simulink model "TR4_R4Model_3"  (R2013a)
settings: Solver=ode23tb  StartTime=0  StopTime=1  FixedStep=1e-4
PreLoadFcn:
  | warning('off','sm:sli:setup:compile:LocalSolverNotSupported')
InitFcn:
  |  SimParam.IC = SM2_InitCondConstrFnc(RawParam,IC);
model workspace (MAT data in the model file):
  handle : class17 (value not decoded)
  handle : class17 (value not decoded)
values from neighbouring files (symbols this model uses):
  RawParam = RobotParamGather(ParamLib)    [main_TR4.m]    (also in DeltaModelMain_v2.m; main_TimeSimulation.m; MGI.m = y)
libraries: SM2_BallJointPartsLib x8, SM2_ForeArmPartsLib x8, SM2_ArmPartsLib x4, SM2_MotorPartsLib x4, ElecDriverLib x1, SM2_FramePartsLib x1, SM2_ToolPartsLib x1

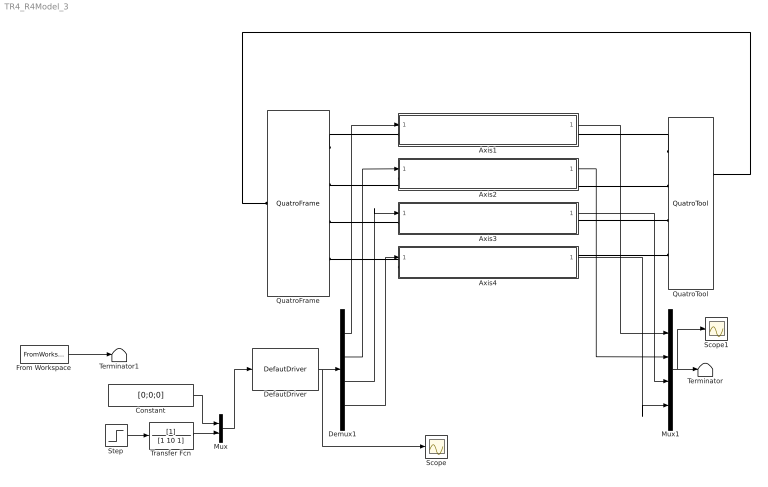
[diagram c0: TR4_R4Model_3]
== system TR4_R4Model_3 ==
  Axis1 : Subsystem
  Axis2 : Subsystem
  Axis3 : Subsystem
  Axis4 : Subsystem
  Constant : Constant  Value=[0;0;0]
  DefautDriver : ElecDriverLib/DefautDriver  VariantControl=driverVarDefault
  Demux1 : Demux
  From Workspace : FromWorkspace  VariableName=simin  SampleTime=0
  Mux : Mux  Inputs=2
  Mux1 : Mux
  QuatroFrame : SM2_FramePartsLib/QuatroFrame
  QuatroTool : SM2_ToolPartsLib/QuatroTool
      link override 6-DOF Joint: ClassName=SixDofJoint  SenseConstraintForceX=off  SenseConstraintForceY=off  SenseConstraintForceZ=off  SenseConstraintTorqueX=off  SenseConstraintTorqueY=off  SenseConstraintTorqueZ=off  ConstraintWrenchDir=FollowerOnBase  ConstraintWrenchFrame=BaseFrame  PxEquilibriumPosition=0  PxEquilibriumPositionUnits=m  PxSpringStiffness=0  PxSpringStiffnessUnits=N/m  PxDampingCoefficient=0  PxDampingCoefficientUnits=N/(m/s)  PxActuationMode=NoActuation  PxSensePosition=off  PxSenseVelocity=off  PxSenseAcceleration=off  PxSenseTorqueForce=off  PxPositionTargetValue=0  PxPositionTargetValueUnits=m  PxPositionTargetSpecify=on  PxPositionTargetPriority=Low  PxVelocityTargetValue=0  PxVelocityTargetValueUnits=m/s  PxVelocityTargetSpecify=on  PxVelocityTargetPriority=High  PyEquilibriumPosition=0  PyEquilibriumPositionUnits=m  PySpringStiffness=0  PySpringStiffnessUnits=N/m  PyDampingCoefficient=0  PyDampingCoefficientUnits=N/(m/s)  PyActuationMode=NoActuation  PySensePosition=off  PySenseVelocity=off  PySenseAcceleration=off  PySenseTorqueForce=off  PyPositionTargetValue=0  PyPositionTargetValueUnits=m  PyPositionTargetSpecify=on  PyPositionTargetPriority=Low  PyVelocityTargetValue=0  PyVelocityTargetValueUnits=m/s  PyVelocityTargetSpecify=on  PyVelocityTargetPriority=High  PzEquilibriumPosition=0  PzEquilibriumPositionUnits=m  PzSpringStiffness=0  PzSpringStiffnessUnits=N/m  PzDampingCoefficient=0  PzDampingCoefficientUnits=N/(m/s)  PzActuationMode=NoActuation  PzSensePosition=off  PzSenseVelocity=off  PzSenseAcceleration=off  PzSenseTorqueForce=off  PzPositionTargetValue=0  PzPositionTargetValueUnits=m  PzPositionTargetSpecify=on  PzPositionTargetPriority=Low  PzVelocityTargetValue=0  PzVelocityTargetValueUnits=m/s  PzVelocityTargetSpecify=on  PzVelocityTargetPriority=High  SphDefPosRotationMethod=None  SphDefPosRotationAngleUnits=deg  SphDefPosRotationStandardAxis=+Z  SphDefPosRotationAngle=0  SphDefPosRotationArbitraryAxis=[0 0 1]  SphDefPosFollAlignAxisA=+X  SphDefPosBaseAlignAxisA=+Y  SphDefPosFollAlignAxisB=+Y  SphDefPosBaseAlignAxisB=+Z  SphEqPosRotationMethod=None  SphEqPosRotationAngleUnits=deg  SphEqPosRotationStandardAxis=+Z  SphEqPosRotationAngle=0  SphEqPosRotationArbitraryAxis=[0 0 1]  SphEqPosFollAlignAxisA=+X  SphEqPosBaseAlignAxisA=+Y  SphEqPosFollAlignAxisB=+Y  SphEqPosBaseAlignAxisB=+Z  SphSpringStiffness=0  SphSpringStiffnessUnits=N*m/deg  SphDampingCoefficient=0  SphDampingCoefficientUnits=N*m/(deg/s)  SphActuateTorqueX=off  SphActuateTorqueY=off  SphActuateTorqueZ=off  SphActuateTorque=off  SphActuationMode=NoActuation  SphActuationFrame=BaseFrame  SphSensePosition=off  SphSenseVelocityX=off  SphSenseVelocityY=off  SphSenseVelocityZ=off  SphSenseVelocity=off  SphSenseAccelerationX=off  SphSenseAccelerationY=off  SphSenseAccelerationZ=off  SphSenseAcceleration=off  SphSenseTorqueX=off  SphSenseTorqueY=off  SphSenseTorqueZ=off  SphSenseTorqueForce=off  SphSensingFrame=BaseFrame  SphPositionTargetRotationMethod=AlignedAxes  SphPositionTargetRotationAngleUnits=deg  SphPositionTargetRotationStandardAxis=+Z  SphPositionTargetRotationAngle=0  SphPositionTargetRotationArbitraryAxis=[0 0 1]  SphPositionTargetFollAlignAxisA=+X  SphPositionTargetBaseAlignAxisA=+X  SphPositionTargetFollAlignAxisB=+Y  SphPositionTargetBaseAlignAxisB=+Y  SphPositionTargetSpecify=on  SphPositionTargetPriority=High  SphVelocityTargetValue=[0 0 0]  SphVelocityTargetValueUnits=deg/s  SphVelocityTargetSpecify=on  SphVelocityTargetPriority=High  SphVelocityTargetInFollowerFrame=on  BlockFunction=simmechanics.library.joints.sixdof_joint
  Scope : Scope
  Scope1 : Scope
  Step : Step  Time=0.01  SampleTime=0
  Terminator : Terminator
  Terminator1 : Terminator
  Transfer Fcn : TransferFcn  Denominator=[1 10 1]
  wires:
  Axis1/1(Alpha) -> Mux1/1
  Axis2/1(Alpha) -> Mux1/2
  Axis4/1(Alpha) -> Mux1/4
  Axis3/1(Alpha) -> Mux1/3
  From Workspace/1 -> Terminator1/1
  DefautDriver/1 -> Scope/1, Demux1/1
  Demux1/1 -> Axis1/1(Torque)
  Demux1/2 -> Axis2/1(Torque)
  Demux1/3 -> Axis3/1(Torque)
  Demux1/4 -> Axis4/1(Torque)
  Mux1/1 -> Scope1/1, Terminator/1
  Step/1 -> Transfer Fcn/1
  Mux/1 -> DefautDriver/1
  Constant/1 -> Mux/1
  Transfer Fcn/1 -> Mux/2
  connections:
  QuatroFrame/RConn1 -- Axis1/LConn1
  Axis2/LConn1 -- QuatroFrame/RConn2
  Axis3/LConn1 -- QuatroFrame/RConn3
  Axis3/RConn1 -- QuatroTool/RConn3
  Axis2/RConn1 -- QuatroTool/RConn2
  QuatroTool/RConn1 -- Axis1/RConn1
  QuatroFrame/LConn1 -- QuatroTool/LConn1
  Axis4/LConn1 -- QuatroFrame/RConn4
  Axis4/RConn1 -- QuatroTool/RConn4

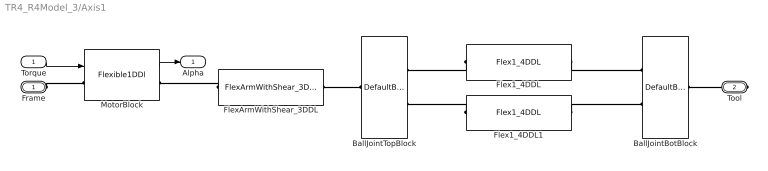
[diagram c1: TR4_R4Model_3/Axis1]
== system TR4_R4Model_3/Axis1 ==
  Torque : Inport
  BallJointBotBlock : SM2_BallJointPartsLib/DefaultBallJointBotPair
  BallJointTopBlock : SM2_BallJointPartsLib/DefaultBallJointTopPair
  Flex1_4DDL : SM2_ForeArmPartsLib/Flex1_4DDL  VariantControl=foreArmVarFlex1_4ddl
  Flex1_4DDL1 : SM2_ForeArmPartsLib/Flex1_4DDL  VariantControl=foreArmVarFlex1_4ddl
  FlexArmWithShear_3DDL : SM2_ArmPartsLib/FlexArmWithShear_3DDL  VariantControl=armVarFlex1_2ddl
  MotorBlock : SM2_MotorPartsLib/Flexible1DDl  VariantControl=motorVarFlex1
      link override Revolute Joint: ClassName=RevoluteJoint  SenseConstraintForceX=off  SenseConstraintForceY=off  SenseConstraintForceZ=off  SenseConstraintTorqueX=off  SenseConstraintTorqueY=off  SenseConstraintTorqueZ=off  ConstraintWrenchDir=FollowerOnBase  ConstraintWrenchFrame=BaseFrame  EquilibriumPosition=SimParam.Motor.Alpha(AxisID)  EquilibriumPositionUnits=rad  SpringStiffness=SimParam.Motor.kSup  SpringStiffnessUnits=N*m/rad  DampingCoefficient=SimParam.Motor.c  DampingCoefficientUnits=N*m/(rad/s)  ActuationMode=TorqueForceActuation  SensePosition=on  SenseVelocity=off  SenseAcceleration=off  SenseTorqueForce=off  PositionTargetValue=SimParam.Motor.Alpha(AxisID)  PositionTargetValueUnits=rad  PositionTargetSpecify=on  PositionTargetPriority=Low  VelocityTargetValue=0  VelocityTargetValueUnits=rad/s  VelocityTargetSpecify=on  VelocityTargetPriority=High  BlockFunction=simmechanics.library.joints.revolute_joint
  Frame : PMIOPort  Port=1  Side=Left
  Tool : PMIOPort  Port=2  Side=Right
  Alpha : Outport
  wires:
  Torque/1 -> MotorBlock/1
  MotorBlock/1 -> Alpha/1
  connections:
  FlexArmWithShear_3DDL/LConn1 -- MotorBlock/RConn1
  Frame/RConn1 -- MotorBlock/LConn1
  FlexArmWithShear_3DDL/RConn1 -- BallJointTopBlock/RConn1
  Tool/RConn1 -- BallJointBotBlock/RConn1
  Flex1_4DDL1/LConn1 -- BallJointTopBlock/LConn2
  Flex1_4DDL/LConn1 -- BallJointTopBlock/LConn1
  Flex1_4DDL/RConn1 -- BallJointBotBlock/LConn1
  Flex1_4DDL1/RConn1 -- BallJointBotBlock/LConn2

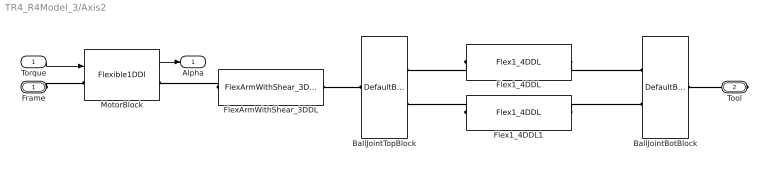
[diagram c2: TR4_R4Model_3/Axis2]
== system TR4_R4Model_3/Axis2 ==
  Torque : Inport
  BallJointBotBlock : SM2_BallJointPartsLib/DefaultBallJointBotPair
  BallJointTopBlock : SM2_BallJointPartsLib/DefaultBallJointTopPair
  Flex1_4DDL : SM2_ForeArmPartsLib/Flex1_4DDL  VariantControl=foreArmVarFlex1_4ddl
  Flex1_4DDL1 : SM2_ForeArmPartsLib/Flex1_4DDL  VariantControl=foreArmVarFlex1_4ddl
  FlexArmWithShear_3DDL : SM2_ArmPartsLib/FlexArmWithShear_3DDL  VariantControl=armVarFlex1_2ddl
  MotorBlock : SM2_MotorPartsLib/Flexible1DDl  VariantControl=motorVarFlex1
      link override Revolute Joint: ClassName=RevoluteJoint  SenseConstraintForceX=off  SenseConstraintForceY=off  SenseConstraintForceZ=off  SenseConstraintTorqueX=off  SenseConstraintTorqueY=off  SenseConstraintTorqueZ=off  ConstraintWrenchDir=FollowerOnBase  ConstraintWrenchFrame=BaseFrame  EquilibriumPosition=SimParam.Motor.Alpha(AxisID)  EquilibriumPositionUnits=rad  SpringStiffness=SimParam.Motor.kSup  SpringStiffnessUnits=N*m/rad  DampingCoefficient=SimParam.Motor.c  DampingCoefficientUnits=N*m/(rad/s)  ActuationMode=TorqueForceActuation  SensePosition=on  SenseVelocity=off  SenseAcceleration=off  SenseTorqueForce=off  PositionTargetValue=SimParam.Motor.Alpha(AxisID)  PositionTargetValueUnits=rad  PositionTargetSpecify=on  PositionTargetPriority=Low  VelocityTargetValue=0  VelocityTargetValueUnits=rad/s  VelocityTargetSpecify=on  VelocityTargetPriority=High  BlockFunction=simmechanics.library.joints.revolute_joint
  Frame : PMIOPort  Port=1  Side=Left
  Tool : PMIOPort  Port=2  Side=Right
  Alpha : Outport
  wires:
  Torque/1 -> MotorBlock/1
  MotorBlock/1 -> Alpha/1
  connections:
  FlexArmWithShear_3DDL/LConn1 -- MotorBlock/RConn1
  Frame/RConn1 -- MotorBlock/LConn1
  FlexArmWithShear_3DDL/RConn1 -- BallJointTopBlock/RConn1
  Tool/RConn1 -- BallJointBotBlock/RConn1
  Flex1_4DDL1/LConn1 -- BallJointTopBlock/LConn2
  Flex1_4DDL/LConn1 -- BallJointTopBlock/LConn1
  Flex1_4DDL/RConn1 -- BallJointBotBlock/LConn1
  Flex1_4DDL1/RConn1 -- BallJointBotBlock/LConn2

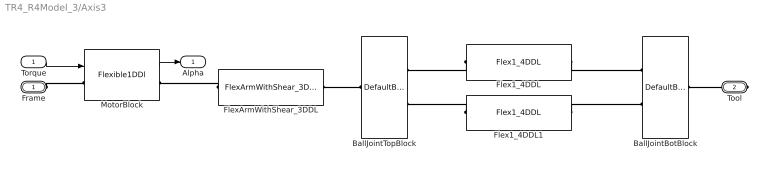
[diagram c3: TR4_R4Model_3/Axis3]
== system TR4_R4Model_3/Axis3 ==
  Torque : Inport
  BallJointBotBlock : SM2_BallJointPartsLib/DefaultBallJointBotPair
  BallJointTopBlock : SM2_BallJointPartsLib/DefaultBallJointTopPair
  Flex1_4DDL : SM2_ForeArmPartsLib/Flex1_4DDL  VariantControl=foreArmVarFlex1_4ddl
  Flex1_4DDL1 : SM2_ForeArmPartsLib/Flex1_4DDL  VariantControl=foreArmVarFlex1_4ddl
  FlexArmWithShear_3DDL : SM2_ArmPartsLib/FlexArmWithShear_3DDL  VariantControl=armVarFlex1_2ddl
  MotorBlock : SM2_MotorPartsLib/Flexible1DDl  VariantControl=motorVarFlex1
      link override Revolute Joint: ClassName=RevoluteJoint  SenseConstraintForceX=off  SenseConstraintForceY=off  SenseConstraintForceZ=off  SenseConstraintTorqueX=off  SenseConstraintTorqueY=off  SenseConstraintTorqueZ=off  ConstraintWrenchDir=FollowerOnBase  ConstraintWrenchFrame=BaseFrame  EquilibriumPosition=SimParam.Motor.Alpha(AxisID)  EquilibriumPositionUnits=rad  SpringStiffness=SimParam.Motor.kSup  SpringStiffnessUnits=N*m/rad  DampingCoefficient=SimParam.Motor.c  DampingCoefficientUnits=N*m/(rad/s)  ActuationMode=TorqueForceActuation  SensePosition=on  SenseVelocity=off  SenseAcceleration=off  SenseTorqueForce=off  PositionTargetValue=SimParam.Motor.Alpha(AxisID)  PositionTargetValueUnits=rad  PositionTargetSpecify=on  PositionTargetPriority=Low  VelocityTargetValue=0  VelocityTargetValueUnits=rad/s  VelocityTargetSpecify=on  VelocityTargetPriority=High  BlockFunction=simmechanics.library.joints.revolute_joint
  Frame : PMIOPort  Port=1  Side=Left
  Tool : PMIOPort  Port=2  Side=Right
  Alpha : Outport
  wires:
  Torque/1 -> MotorBlock/1
  MotorBlock/1 -> Alpha/1
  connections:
  FlexArmWithShear_3DDL/LConn1 -- MotorBlock/RConn1
  Frame/RConn1 -- MotorBlock/LConn1
  FlexArmWithShear_3DDL/RConn1 -- BallJointTopBlock/RConn1
  Tool/RConn1 -- BallJointBotBlock/RConn1
  Flex1_4DDL1/LConn1 -- BallJointTopBlock/LConn2
  Flex1_4DDL/LConn1 -- BallJointTopBlock/LConn1
  Flex1_4DDL/RConn1 -- BallJointBotBlock/LConn1
  Flex1_4DDL1/RConn1 -- BallJointBotBlock/LConn2

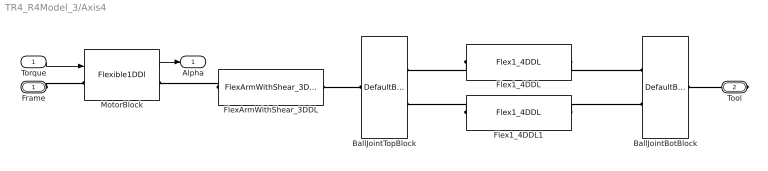
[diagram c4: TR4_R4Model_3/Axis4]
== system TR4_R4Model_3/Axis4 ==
  Torque : Inport
  BallJointBotBlock : SM2_BallJointPartsLib/DefaultBallJointBotPair
  BallJointTopBlock : SM2_BallJointPartsLib/DefaultBallJointTopPair
  Flex1_4DDL : SM2_ForeArmPartsLib/Flex1_4DDL  VariantControl=foreArmVarFlex1_4ddl
  Flex1_4DDL1 : SM2_ForeArmPartsLib/Flex1_4DDL  VariantControl=foreArmVarFlex1_4ddl
  FlexArmWithShear_3DDL : SM2_ArmPartsLib/FlexArmWithShear_3DDL  VariantControl=armVarFlex1_2ddl
  MotorBlock : SM2_MotorPartsLib/Flexible1DDl  VariantControl=motorVarFlex1
      link override Revolute Joint: ClassName=RevoluteJoint  SenseConstraintForceX=off  SenseConstraintForceY=off  SenseConstraintForceZ=off  SenseConstraintTorqueX=off  SenseConstraintTorqueY=off  SenseConstraintTorqueZ=off  ConstraintWrenchDir=FollowerOnBase  ConstraintWrenchFrame=BaseFrame  EquilibriumPosition=SimParam.Motor.Alpha(AxisID)  EquilibriumPositionUnits=rad  SpringStiffness=SimParam.Motor.kSup  SpringStiffnessUnits=N*m/rad  DampingCoefficient=SimParam.Motor.c  DampingCoefficientUnits=N*m/(rad/s)  ActuationMode=TorqueForceActuation  SensePosition=on  SenseVelocity=off  SenseAcceleration=off  SenseTorqueForce=off  PositionTargetValue=SimParam.Motor.Alpha(AxisID)  PositionTargetValueUnits=rad  PositionTargetSpecify=on  PositionTargetPriority=Low  VelocityTargetValue=0  VelocityTargetValueUnits=rad/s  VelocityTargetSpecify=on  VelocityTargetPriority=High  BlockFunction=simmechanics.library.joints.revolute_joint
  Frame : PMIOPort  Port=1  Side=Left
  Tool : PMIOPort  Port=2  Side=Right
  Alpha : Outport
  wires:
  Torque/1 -> MotorBlock/1
  MotorBlock/1 -> Alpha/1
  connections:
  FlexArmWithShear_3DDL/LConn1 -- MotorBlock/RConn1
  Frame/RConn1 -- MotorBlock/LConn1
  FlexArmWithShear_3DDL/RConn1 -- BallJointTopBlock/RConn1
  Tool/RConn1 -- BallJointBotBlock/RConn1
  Flex1_4DDL1/LConn1 -- BallJointTopBlock/LConn2
  Flex1_4DDL/LConn1 -- BallJointTopBlock/LConn1
  Flex1_4DDL/RConn1 -- BallJointBotBlock/LConn1
  Flex1_4DDL1/RConn1 -- BallJointBotBlock/LConn2
